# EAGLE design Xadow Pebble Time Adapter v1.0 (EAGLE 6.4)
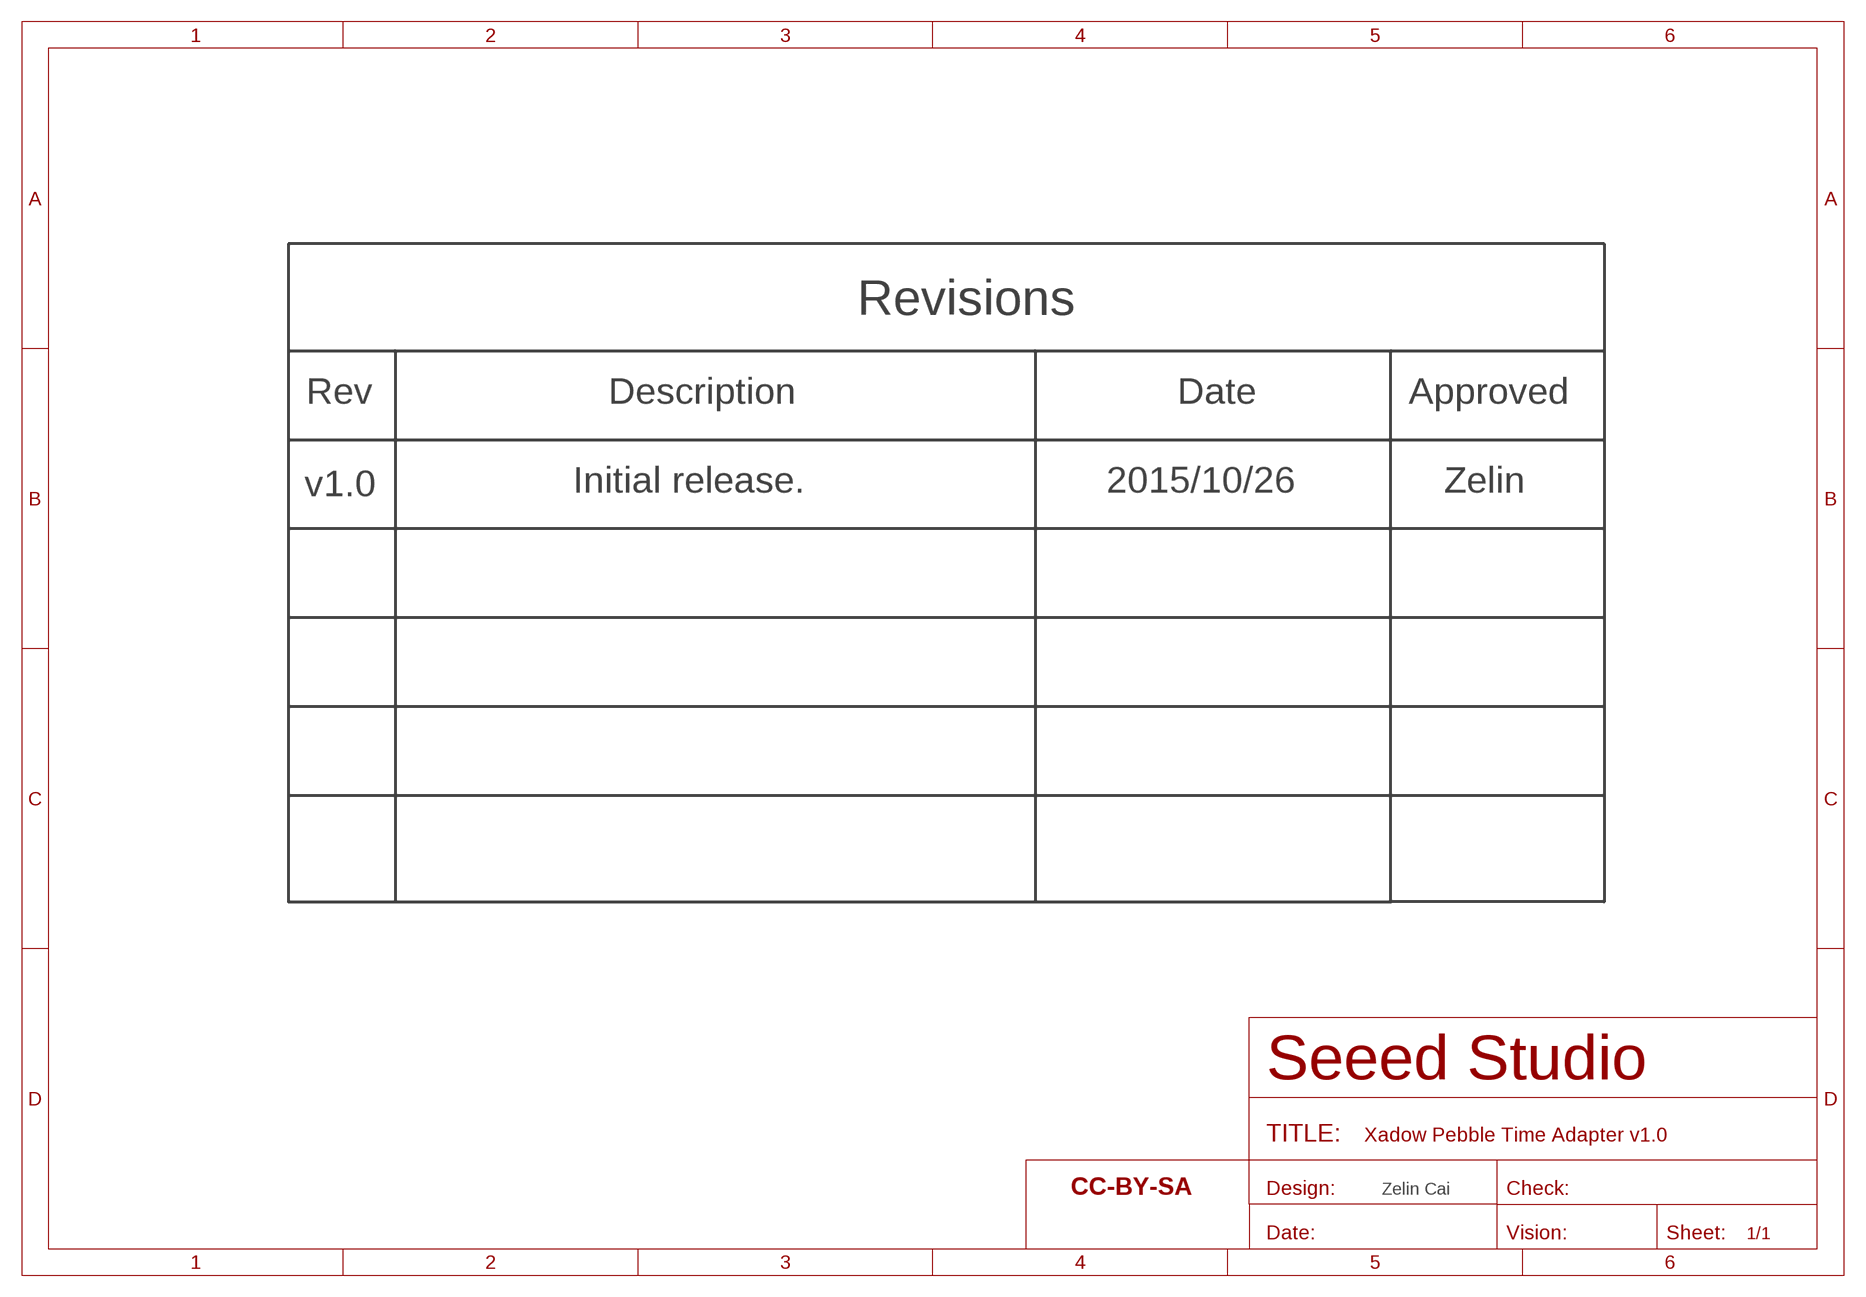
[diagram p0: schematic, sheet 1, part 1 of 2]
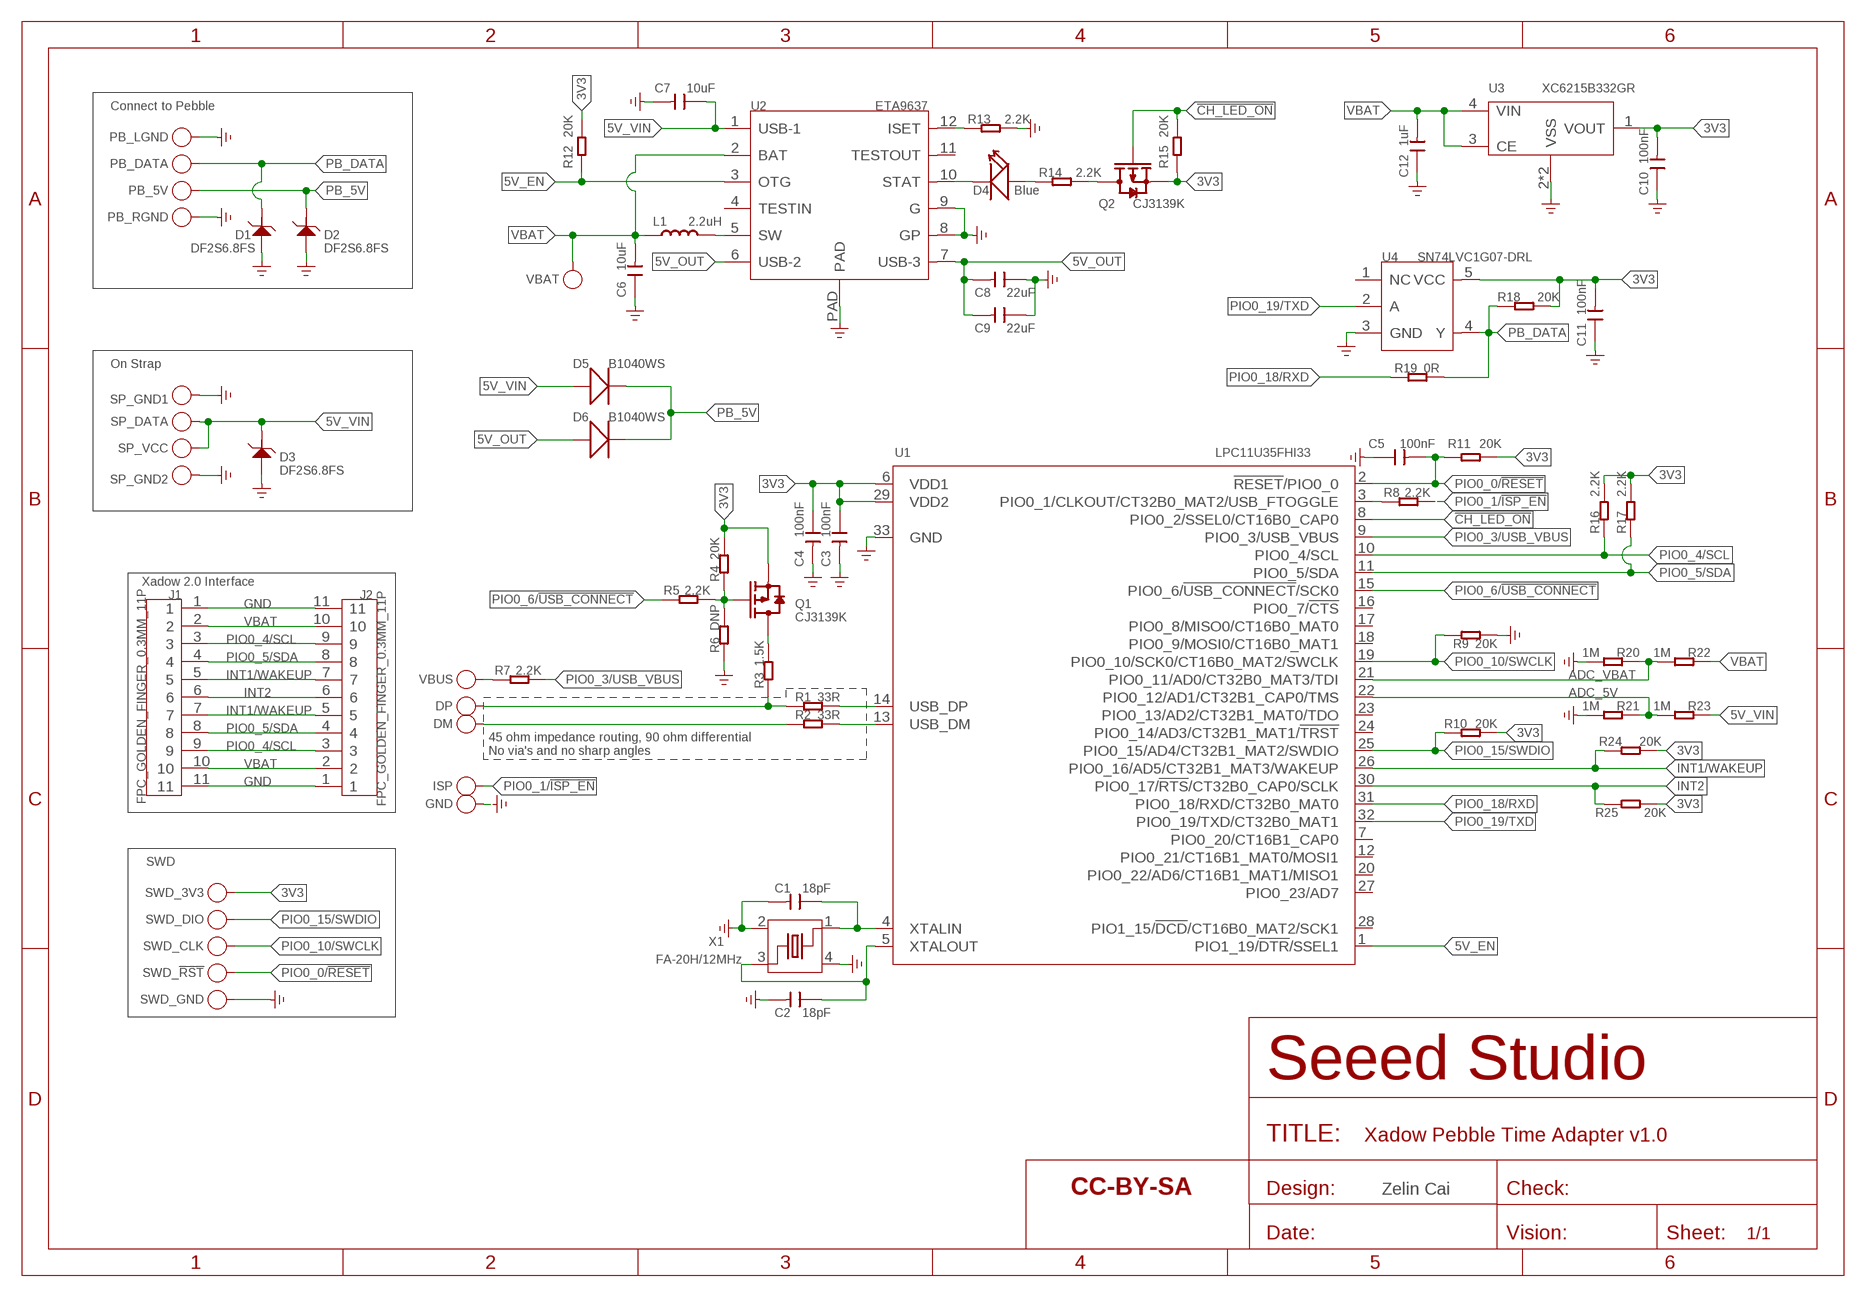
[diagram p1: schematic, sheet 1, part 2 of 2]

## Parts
C1  18pF  CAP-0201  [C0201]
C2  18pF  CAP-0201  [C0201]
C3  100nF  CAP-0201  [C0201]
C4  100nF  CAP-0201  [C0201]
C5  100nF  CAP-0201  [C0201]
C6  10uF  CAP-0805  [C0805]
C7  10uF  CAP-0805  [C0805]
C8  22uF  CAP-0805  [C0805]
C9  22uF  CAP-0805  [C0805]
C10  100nF  CAP-0201  [C0201]
C11  100nF  CAP-0201  [C0201]
C12  1uF  CAP-0402  [C0402]
D1  DF2S6.8FS  D-ESD-2P'DF2S6.8FS'  [SOD-923]
D2  DF2S6.8FS  D-ESD-2P'DF2S6.8FS'  [SOD-923]
D3  DF2S6.8FS  D-ESD-2P'DF2S6.8FS'  [SOD-923]
D4  Blue  LED'0402'  [LED-0402]
D5  B1040WS  DIODE'0805'  [SOD-323]
D6  B1040WS  DIODE'0805'  [SOD-323]
DM  DM  TEST-POINT'4545'  [TP-D45MIL]
DP  DP  TEST-POINT'4545'  [TP-D45MIL]
FR1  PAGE1  SEEEDSTUDIO-OPEN-SCH-FRAME  [SEEEDSTUDIO-PCB-FRAME]
FR2  PAGE2  SEEEDSTUDIO-OPEN-SCH-FRAME  [SEEEDSTUDIO-PCB-FRAME]
GND  GND  TEST-POINT'4545'  [TP-D45MIL]
ISP  ISP  TEST-POINT'4545'  [TP-D45MIL]
J1  FPC_GOLDEN_FINGER_0.3MM_11P  FPC-GOLDFINGER-11(FH35C-11S-0.3SHW(50))  [FPC_GOLDEN_FINGER_0.3MM_11P(FH35C-11S-0.3SHW(50))]
J2  FPC_GOLDEN_FINGER_0.3MM_11P  FPC-GOLDFINGER-11(FH35C-11S-0.3SHW(50))  [FPC_GOLDEN_FINGER_0.3MM_11P(FH35C-11S-0.3SHW(50))]
L1  2.2uH  INDUCTOR/FERRITE-BEAD'0806'  [L0806]
PB_5V  Pogo_M014  POGO-PIN-86  [TP-D86MIL$1]
PB_DATA  Pogo_M014  POGO-PIN-86  [TP-D86MIL$1]
PB_LGND  Pogo_M041  POGO-PIN-100  [TP-D100MIL]
PB_RGND  Pogo_M041  POGO-PIN-100  [TP-D100MIL]
Q1  CJ3139K  MOSFET-P-CJ3139K  [SOT-723]
Q2  CJ3139K  MOSFET-P-CJ3139K  [SOT-723]
R1  33R  RES-0201  [R0201]
R2  33R  RES-0201  [R0201]
R3  1.5K  RES-0201  [R0201]
R4  20K  RES-0201  [R0201]
R5  2.2K  RES-0201  [R0201]
R6  DNP  RES-0201  [R0201]
R7  2.2K  RES-0201  [R0201]
R8  2.2K  RES-0201  [R0201]
R9  20K  RES-0201  [R0201]
R10  20K  RES-0201  [R0201]
R11  20K  RES-0201  [R0201]
R12  20K  RES-0201  [R0201]
R13  2.2K  RES-0201  [R0201]
R14  2.2K  RES-0201  [R0201]
R15  20K  RES-0201  [R0201]
R16  2.2K  RES-0201  [R0201]
R17  2.2K  RES-0201  [R0201]
R18  20K  RES-0201  [R0201]
R19  0R  RES-0201  [R0201]
R20  1M  RES-0201  [R0201]
R21  1M  RES-0201  [R0201]
R22  1M  RES-0201  [R0201]
R23  1M  RES-0201  [R0201]
R24  20K  RES-0201  [R0201]
R25  20K  RES-0201  [R0201]
SP_DATA  5V_VIN  POGO-PIN-86  [TP-D86MIL$1]
SP_GND1  GND  POGO-PIN-1-2.0MM  [TP-D2.0MM]
SP_GND2  GND  POGO-PIN-1-2.0MM  [TP-D2.0MM]
SP_VCC  5V_VIN  POGO-PIN-86  [TP-D86MIL$1]
SWD_3V3  SWD_3V3  TEST-POINT'4545'  [TP-D45MIL]
SWD_!RST  SWD_!RST  TEST-POINT'4545'  [TP-D45MIL]
SWD_CLK  SWD_CLK  TEST-POINT'4545'  [TP-D45MIL]
SWD_DIO  SWD_DIO  TEST-POINT'4545'  [TP-D45MIL]
SWD_GND  SWD_GND  TEST-POINT'4545'  [TP-D45MIL]
U1  LPC11U35FHI33  MCU-LPC11U35FHI33/501  [QFN32G-0.5-5X5MM]
U2  ETA9637  PMIC-ETA9637  [QFN12-0.45-3X3MM]
U3  XC6215B332GR  PMIC-XC6215-3V3  [USP4-0.6-1.2X1.6MM]
U4  SN74LVC1G07-DRL  LOGIC-SN74LVC1G07-DRL  [5P-SDM-1.6X1.2X0.5MM]
VBAT  VBAT  TEST-POINT'4545'  [TP-D45MIL]
VBUS  VBUS  TEST-POINT'4545'  [TP-D45MIL]
X1  FA-20H/12MHz  CRYSTAL'NX2520SA'  [X4-SMD-2.5X2.0X0.8MM]

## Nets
3V3: C3.1 C4.1 C10.2 C11.2 Q1.3(S) Q2.3(S) R4.2 R10.2 R11.1 R12.2 R15.1 R16.1 R17.1 R18.2 R24.1 R25.2 SWD_3V3.T U1.6(VDD1) U1.29(VDD2) U3.1(VOUT) U4.5(VCC)
5V_EN: R12.1 U1.1(PIO1_19/!DTR!/SSEL1) U2.3(OTG)
5V_OUT: C8.2 C9.2 D6.+ U2.6(USB-2) U2.7(USB-3)
5V_VIN: C7.1 D3.1 D5.+ R23.1 SP_DATA.T SP_VCC.T U2.1(USB-1)
!CH_LED_ON: Q2.1(G) R15.2 U1.8(PIO0_2/SSEL0/CT16B0_CAP0)
ADC_5V: R21.1 R23.2 U1.22(PIO0_12/AD1/CT32B1_CAP0/TMS)
ADC_VBAT: R20.1 R22.2 U1.21(PIO0_11/AD0/CT32B0_MAT3/TDI)
GND: C1.2 C2.2 C3.2 C4.2 C5.1 C6.1 C7.2 C8.1 C9.1 C10.1 C11.1 C12.1 D1.2 D2.2 D3.2 GND.T J1.1 J1.11 J2.1 J2.11 PB_LGND.T PB_RGND.T R6.1 R9.2 R13.1 R20.2 R21.2 SP_GND1.T SP_GND2.T SWD_GND.T U1.33(GND) U2.8(GP) U2.9(G) U2.PAD U3.2(VSS) U3.PAD(VSS) U4.3(GND) X1.2 X1.4 ; supply symbol labelled GND_POWER
INT1/WAKEUP: J1.5 J1.7 J2.5 J2.7 R24.2 U1.26(PIO0_16/AD5/CT32B1_MAT3/WAKEUP)
INT2: J1.6 J2.6 R25.1 U1.30(PIO0_17/!RTS!/CT32B0_CAP0/SCLK)
N$1: C1.1 U1.4(XTALIN) X1.1
N$2: Q1.2(D) R3.2
N$3: C2.1 U1.5(XTALOUT) X1.3
N$4: R1.2 U1.14(USB_DP)
N$5: R2.2 U1.13(USB_DM)
N$6: DP.T R1.1 R3.1
N$7: Q1.1(G) R4.1 R5.1 R6.2
N$8: DM.T R2.1
N$9: R7.2 VBUS.T
N$10: R8.2 U1.3(PIO0_1/CLKOUT/CT32B0_MAT2/USB_FTOGGLE)
N$11: L1.2 U2.5(SW)
N$12: R13.2 U2.12(ISET)
N$13: D4.- U2.10(STAT)
N$14: D4.+ R14.2
N$15: Q2.2(D) R14.1
PB_5V: D2.1 D5.- D6.- PB_5V.T
PB_DATA: D1.1 PB_DATA.T R18.1 R19.1 U4.4(Y)
PIO0_0/!RESET: C5.2 R11.2 SWD_!RST.T U1.2(!RESET!/PIO0_0)
PIO0_1/!ISP_EN: ISP.T R8.1
PIO0_3/USB_VBUS: R7.1 U1.9(PIO0_3/USB_VBUS)
PIO0_4/SCL: J1.3 J1.9 J2.3 J2.9 R16.2 U1.10(PIO0_4/SCL)
PIO0_5/SDA: J1.4 J1.8 J2.4 J2.8 R17.2 U1.11(PIO0_5/SDA)
PIO0_6/!USB_CONNECT: R5.2 U1.15(PIO0_6/!USB_CONNECT!/SCK0)
PIO0_10/SWCLK: R9.1 SWD_CLK.T U1.19(PIO0_10/SCK0/CT16B0_MAT2/SWCLK)
PIO0_15/SWDIO: R10.1 SWD_DIO.T U1.25(PIO0_15/AD4/CT32B1_MAT2/SWDIO)
PIO0_18/RXD: R19.2 U1.31(PIO0_18/RXD/CT32B0_MAT0)
PIO0_19/TXD: U1.32(PIO0_19/TXD/CT32B0_MAT1) U4.2(A)
VBAT: C6.2 C12.2 J1.2 J1.10 J2.2 J2.10 L1.1 R22.1 U2.2(BAT) U3.3(CE) U3.4(VIN) VBAT.T
Unconnected: U1.7(PIO0_20/CT16B1_CAP0) U1.12(PIO0_21/CT16B1_MAT0/MOSI1) U1.16(PIO0_7/!CTS!) U1.17(PIO0_8/MISO0/CT16B0_MAT0) U1.18(PIO0_9/MOSI0/CT16B0_MAT1) U1.20(PIO0_22/AD6/CT16B1_MAT1/MISO1) U1.23(PIO0_13/AD2/CT32B1_MAT0/TDO) U1.24(PIO0_14/AD3/CT32B1_MAT1/!TRST!) U1.27(PIO0_23/AD7) U1.28(PIO1_15/!DCD!/CT16B0_MAT2/SCK1) U2.4(TESTIN) U2.11(TESTOUT) U4.1(NC)

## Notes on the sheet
- Connect to Pebble
- Revisions
- On Strap
- Rev | Description | Date | Approved
- v1.0 | Initial release. | 2015/10/26 | Zelin
- Xadow 2.0 Interface
- 45 ohm impedance routing, 90 ohm differential
  No via's and no sharp angles
- SWD
- Zelin Cai | Zelin Cai

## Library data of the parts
C1-C12 = Discrete-new:CAP: Ceramic Capacitors
D1-D3 = Discrete-new:D-ESD-2P: SOD-923:304060009;SOD-123:304060001
D4 = Discrete-new:LED
D5 D6 = Discrete-new:DIODE*
DM DP GND ISP SWD_3V3 SWD_!RST SWD_CLK SWD_DIO SWD_GND VBAT VBUS = Discrete-new:TEST-POINT; PARTNO: DNP
FR1 FR2 = moudle-new:SEEEDSTUDIO-OPEN-SCH-FRAME
J1 J2 = Connector:FPC-GOLDFINGER-11(FH35C-11S-0.3SHW(50))
L1 = Discrete-new:INDUCTOR/FERRITE-BEAD
PB_5V PB_DATA PB_LGND PB_RGND SP_DATA SP_VCC = Connector-new:POGO-PIN
Q1 Q2 = Discrete-new:MOSFET-P
R1-R25 = Discrete-new:RES
SP_GND1 SP_GND2 = Connector-new:POGO-PIN-1
U1 = IC-new:MCU-LPC11U35FHI33/501: 310010053
U2 = template:PMIC-ETA9637: 1.5A Linear Charger with 1A OTG
U3 = IC-new:PMIC-XC6215-3V3
U4 = template:LOGIC-SN74LVC1G07: SN74LVC1G07 Single Buffer/Driver With Open-Drain Output
X1 = Discrete-new:CRYSTAL

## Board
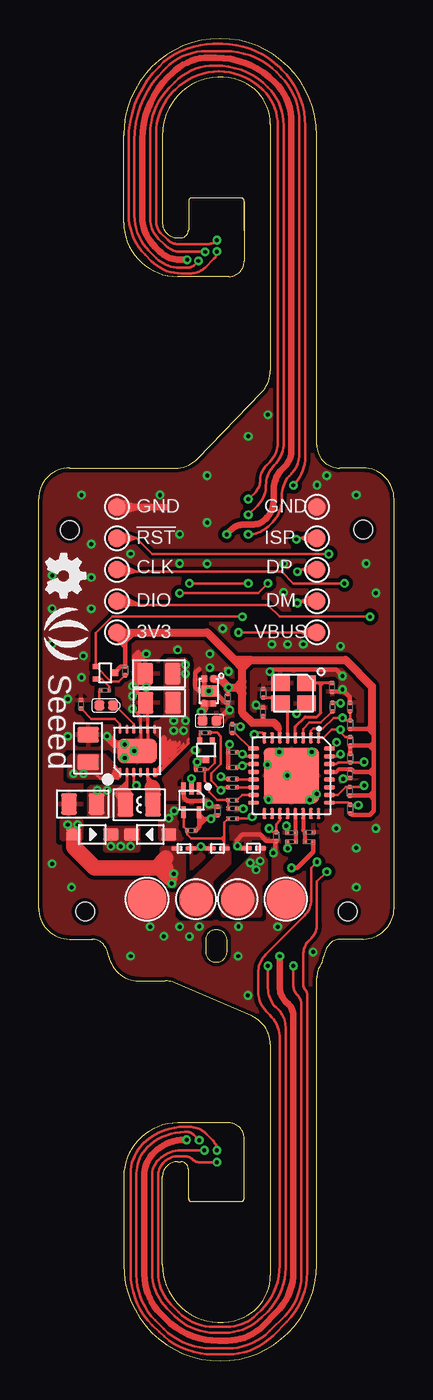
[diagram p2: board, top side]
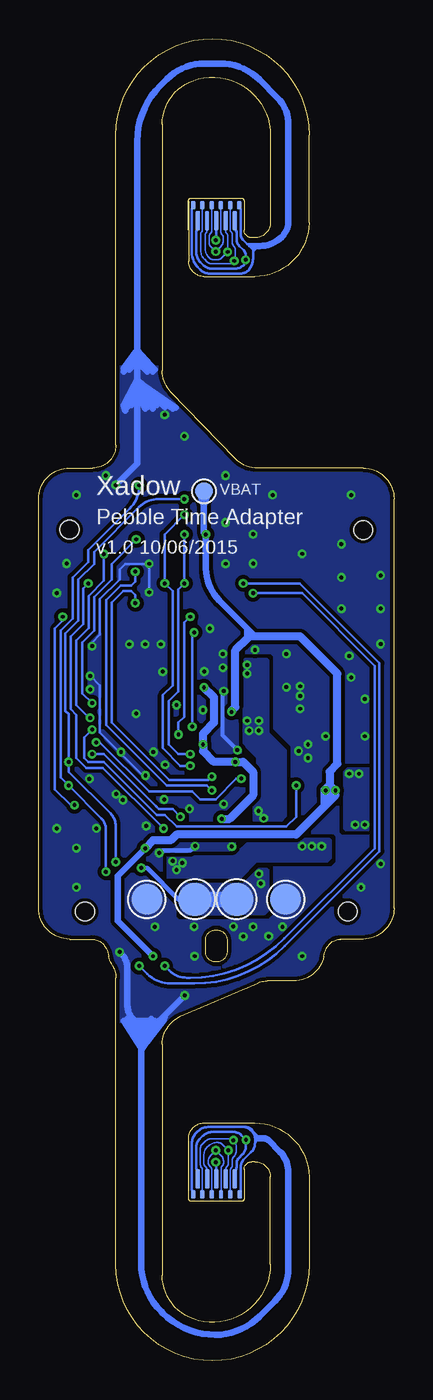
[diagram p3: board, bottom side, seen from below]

Size 23 x 85.6 mm. Coordinates in mm from the lower left corner, seen from the top.
Outline: 58 segments
Copper layers (1*16): Top 0.035mm / dielectric 1.5mm / Bottom 0.035mm
Design rules "SeeedStudio_2layer_DRU_no_angle_20140221 *": minimum track width 1mil, minimum drill 10mil, track to track 6mil, track to pad 6mil, pad to pad 6mil, via to via 6mil, smd to smd 0mil, copper to edge 10mil, drill to drill 10mil, minimum pad ring 10mil, minimum via ring 6mil, stop-mask expansion 2mil, vias tented up to drill 25mil, thermal gap 10mil
Holes 1.2 mm at 20,29.09 3,29.09 21,53.81 2,53.79
tRestrict: 1 lines

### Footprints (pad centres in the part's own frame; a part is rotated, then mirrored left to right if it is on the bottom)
C0201 = smd 0.279 x 0.318: 1 -0.279,0; 2 0.279,0
C0805 = smd 1.397 x 1.016: 1 0,0.889; 2 0,-0.889
C0402 = smd 0.635 x 0.635: 1 0,0.445; 2 0,-0.445
SOD-923 = smd 0.7 x 0.3: 1 -0.45,0; 2 0.45,0
LED-0402 = smd 0.635 x 0.635: + -0.445,0; - 0.445,0
SOD-323 = smd 1 x 0.8: + -1.2,0; - 1.2,0
TP-D45MIL = smd 1.143 x 1.143: T 0,0
FPC_GOLDEN_FINGER_0.3MM_11P(FH35C-11S-0.3SHW(50)) = smd 0.28 x 0.55: 1 -1.5,0; 3 -0.9,0; 5 -0.3,0; 7 0.3,0; 9 0.9,0; 11 1.5,0 | smd 0.28 x 1.25: 2 -1.2,-1; 4 -0.6,-1; 6 0,-1; 8 0.6,-1; 10 1.2,-1
L0806 = smd 1.016 x 1.524: 1 -0.889,0; 2 0.889,0
TP-D86MIL$1 = smd 2.184 x 2.184: T 0,0
TP-D100MIL = smd 2.54 x 2.54: T 0,0
SOT-723 = smd 0.32 x 0.4: 1 -0.4,-0.6; 2 0.4,-0.6 | smd 0.42 x 0.5: 3 0,0.6
R0201 = smd 0.279 x 0.318: 1 -0.279,0; 2 0.279,0
TP-D2.0MM = smd 2 x 2: T 0,0
QFN32G-0.5-5X5MM = smd 0.7 x 0.25: 1 -2.45,1.75; 2 -2.45,1.25; 3 -2.45,0.75; 4 -2.45,0.25; 5 -2.45,-0.25; 6 -2.45,-0.75; 7 -2.45,-1.25; 8 -2.45,-1.75; 17 2.45,-1.75; 18 2.45,-1.25; 19 2.45,-0.75; 20 2.45,-0.25; 21 2.45,0.25; 22 2.45,0.75; 23 2.45,1.25; 24 2.45,1.75 | smd 0.25 x 0.7: 9 -1.75,-2.45; 10 -1.25,-2.45; 11 -0.75,-2.45; 12 -0.25,-2.45; 13 0.25,-2.45; 14 0.75,-2.45; 15 1.25,-2.45; 16 1.75,-2.45; 25 1.75,2.45; 26 1.25,2.45; 27 0.75,2.45; 28 0.25,2.45; 29 -0.25,2.45; 30 -0.75,2.45; 31 -1.25,2.45; 32 -1.75,2.45 | smd 3.6 x 3.6: 33 0,0
QFN12-0.45-3X3MM = smd 0.2 x 0.6: 1 -1.125,-1.4; 2 -0.675,-1.4; 3 -0.225,-1.4; 4 0.225,-1.4; 5 0.675,-1.4; 6 1.125,-1.4; 7 1.125,1.4; 8 0.675,1.4; 9 0.225,1.4; 10 -0.225,1.4; 11 -0.675,1.4; 12 -1.125,1.4 | smd 2.55 x 1.6: PAD 0,0
USP4-0.6-1.2X1.6MM = smd 0.36 x 0.4: 1 -0.3,-0.8; 2 0.3,-0.8; 3 0.3,0.8; 4 -0.3,0.8 | smd 1 x 0.7: PAD 0,0
5P-SDM-1.6X1.2X0.5MM = smd 0.3 x 0.75: 1 -0.5,-0.775; 2 0,-0.775; 3 0.5,-0.775; 4 0.5,0.775; 5 -0.5,0.775
X4-SMD-2.5X2.0X0.8MM = smd 1.2 x 1: 1 -0.85,-0.65; 2 0.85,-0.65; 3 0.85,0.65; 4 -0.85,0.65

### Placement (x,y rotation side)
C1  18.99,43.6 270 top
C2  14.53,43.22 90 top
C3  20.15,38.01 270 top
C4  14.52,42.01 90 top
C5  20.15,42.33 270 top
C6  2.85,36.04 90 top
C7  3.21,39.65 180 top
C8  7.8,42.61 90 top
C9  7.79,44.49 90 top
C10  12.24,42.9 90 top
C11  11.59,35.6 270 top
C12  11.05,41.44 270 top
D1  11.58,33.18 180 top
D2  13.9,33.18 180 top
D3  9.41,33.17 0 top
D4  4.37,42.43 0 top
D5  3.47,34.07 0 top
D6  7.22,34.07 180 top
DM  18.01,49.19 0 top
DP  18.01,51.22 0 top
FR1  not placed on the board
FR2  not placed on the board
GND  18.01,55.28 0 top
ISP  18.01,53.25 0 top
J1  11.5,74.81 0 bottom
J2  11.5,10.79 180 bottom
L1  6.51,36 0 top
PB_5V  12.88,29.88 0 top
PB_DATA  10.19,29.88 0 top
PB_LGND  7.02,29.88 0 top
PB_RGND  15.99,29.88 0 top
Q1  10.84,39.55 180 top
Q2  4.31,44.54 270 top
R1  12.55,37.14 0 top
R2  12.55,37.67 0 top
R3  10.77,40.67 180 top
R4  10.46,38.29 180 top
R5  12.55,36.3 0 top
R6  12.55,35.76 180 top
R7  12.53,40.93 90 top
R8  19.02,42.33 270 top
R9  15.37,33.95 270 top
R10  20.16,35.73 270 top
R11  20.16,41.19 90 top
R12  20.17,40.11 270 top
R13  2.74,42.51 270 top
R14  4.28,43.41 180 top
R15  5.61,44.67 270 top
R16  12.55,39.41 0 top
R17  12.55,38.42 0 top
R18  9.89,34.34 0 top
R19  12.55,35.1 0 top
R20  16.36,34.2 180 top
R21  17.51,34.23 0 top
R22  16.36,33.62 0 top
R23  17.51,33.62 180 top
R24  20.13,36.87 90 top
R25  20.17,39.03 90 top
SP_DATA  10.19,29.88 0 bottom
SP_GND1  7.02,29.88 0 bottom
SP_GND2  15.99,29.88 0 bottom
SP_VCC  12.88,29.88 0 bottom
SWD_3V3  5.06,47.16 180 top
SWD_!RST  5.06,53.25 180 top
SWD_CLK  5.06,51.22 180 top
SWD_DIO  5.06,49.19 180 top
SWD_GND  5.06,55.28 180 top
U1  16.36,37.88 270 top
U2  6.38,39.48 0 top
U3  11.02,43.36 180 top
U4  9.89,36.28 180 top
U$32  [SEEED-SILK-160*153MIL]  1.88,47.03 270 top
U$33  [OSHW_FILLX100_NOTEXT]  0.49,52.24 270 top
VBAT  12.3,56.3 90 bottom
VBUS  18.01,47.16 0 top
X1  16.49,43.22 180 top

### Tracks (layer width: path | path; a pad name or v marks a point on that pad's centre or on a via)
3V3  (via drill 0.25 pad 0.51)
  Top 0.152: 21.57,41.06 21.51,41.12
  Top 0.254: U1.6 15.61,40.92 15.47,41.06 | 14.46,41.31 14.52,41.38 C4.1 14.52,41.63 | 14.52,41.63 14.33,41.44 | 14.52,41.63 14.71,41.44 | U1.29 19.28,38.13 19.44,38.29 C3.1
  Top 0.305: C10.2 12.24,43.54 v12.3,43.6 | U4.5 10.39,35.1 | R4.2 10.18,38.68 v10.27,38.77 10.44,38.95 Q1.3 | R10.2 20.2,35.45 20.3,35.34 21.44,35.34 21.7,35.6 21.7,36.36 | 21.7,36.36 21.7,36.61 | 21.7,36.61 21.7,36.87 | 21.7,36.87 21.7,37.88 | 21.7,37.88 21.7,38.14 | 21.7,38.14 21.7,38.39 | 21.7,38.39 21.7,39.54 | 21.7,39.54 21.7,39.79 | R11.1 21.33,40.91 | 21.34,40.91 21.67,40.91 21.7,40.93 | 21.4,39.83 R12.2 R25.2 | 21.48,39.83 21.66,39.83 21.7,39.79 | C3.1 20.27,38.29 20.43,38.14 21.44,38.14 | 21.44,38.14 21.7,38.14 | R17.1 R16.1 12.27,39.83 v12.36,39.92 | R24.1 21.42,36.59 | 21.47,36.59 21.67,36.59 21.7,36.61 | 21.7,39.79 21.7,40.04 | 21.7,40.04 21.7,40.55 | 21.7,40.55 21.7,40.93 | 21.7,40.93 21.7,41.19 | 21.33,40.91 21.33,40.94 21.51,41.12 21.57,41.19 | 21.33,40.91 21.34,40.91 | 21.34,40.91 21.7,40.55 | 21.4,39.83 21.48,39.83 | 21.48,39.83 21.7,40.04 | 21.4,39.83 21.7,39.54 | 21.44,38.14 21.7,38.39 | 21.44,38.14 21.7,37.88 | 21.42,36.59 21.7,36.87 | 21.42,36.59 21.47,36.59 | 21.47,36.59 21.7,36.36 | C11.2 11.38,35.32 v11.16,35.09 10.77,35.09 | 10.55,34.86 10.55,34.94 10.39,35.09 | 10.65,35.09 10.39,35.09 | 10.39,35.09 10.39,35.1 | 10.77,35.09 10.65,35.09 | 10.65,35.09 10.39,35.34 | 10.77,35.09 10.55,34.86 | 10.39,35.1 10.39,34.56 R18.2 | 10.55,34.86 10.39,34.71 | 5.61,46.23 R15.1 5.32,44.95 Q2.3 | 5.61,46.23 5.61,46.52 | 5.61,46.56 5.61,47.12 5.57,47.16 | 5.61,46.52 5.56,46.52 5.19,46.9 | 5.61,46.52 5.61,46.56 | 5.61,46.56 6.08,47.03 5.19,47.54 | 5.61,46.23 4.93,46.9
  Top 0.508: 12.22,43.52 v12.3,43.6 | v12.3,43.6 12.81,43.6 | 12.81,43.6 13.19,43.6 | 15.47,41.06 15.22,41.31 14.46,41.31 13.82,41.31 13.19,41.95 13.19,43.22 | U3.1 11.74,44.16 v12.3,43.6 | 13.19,43.22 13.19,43.6 | 13.19,43.6 13.19,43.98 | 12.81,43.6 13.19,43.98 | 12.81,43.6 13.19,43.22 | 13.7,45.38 19.86,45.38 21.57,43.67 21.57,41.06 | 13.7,45.38 13.19,45.38 | 13.19,45.38 12.68,45.38 | 13.19,43.98 13.19,44.87 | 13.19,44.87 13.19,45.38 | 13.19,44.87 12.68,45.38 | 13.19,44.87 13.7,45.38 | 12.68,45.38 10.9,47.16 5.57,47.16 SWD_3V3.T
  Bottom 0.508: v12.3,43.6 11.66,42.96 11.66,41.31 12.36,40.61 v12.36,39.92 12.36,39.47 11.66,38.77 v10.27,38.77 9.76,38.77 9.12,38.14 9.12,36.61 10.65,35.09 v11.16,35.09
5V_EN  (via drill 0.25 pad 0.51)
  Top 0.152: U2.3 6.16,37.42 v6.33,37.25 | U1.1 18.43,40.33 18.97,40.87 v19.54,40.87 19.54,40.68 19.83,40.39 R12.1
  Bottom 0.152: v19.54,40.87 20.05,40.36 20.05,39.03 19.79,38.77 18.78,38.77 15.35,35.34 14.84,35.34 14.08,34.58 6.96,34.58 6.33,35.22 v6.33,37.25
5V_OUT  (via drill 0.25 pad 0.51)
  Top 0.203: 8.23,38.9 8.11,38.77 7.51,38.17 U2.6 7.67,38.08 | 8.23,38.9 8.49,39.15 8.49,40.17 | 7.67,38.08 8.49,38.9 | 7.67,38.08 7.6,38.01 7.54,38.01 | 8.49,38.9 8.49,38.77 | 8.49,38.77 7.6,37.88 7.54,37.88 | 8.49,38.9 8.62,39.03 | 8.62,39.03 8.74,39.15 | 8.74,39.15 8.74,40.04 | 8.49,38.77 8.87,39.15 | 8.87,39.15 8.87,39.41 | 8.87,39.66 8.87,39.79 | 8.87,39.79 8.87,40.04 | 8.62,39.03 8.62,39.66 | 8.62,39.66 8.62,40.04 | 8.62,39.66 8.36,39.92 | 8.87,39.79 9.12,40.04 | 8.23,38.9 8.36,38.9 8.36,40.04 | 8.74,39.15 8.87,39.15 | 8.87,39.15 9.7,39.98 9.7,40.23 | 8.87,39.41 9.38,39.92 | 8.87,39.41 8.87,39.66 | 8.87,39.66 9.12,39.92
  Top 0.406: 8.11,38.77 8.11,40.3
  other vias: 9.5,45.06 9.5,44.49 8.43,35.13 8.77,35.6 9.5,41.44 8.74,41.44 8.74,40.81 9.38,40.81
  pour Top (isolate 0.254, no thermals): 8.11,33.69 9.25,33.69 9.38,33.82 9.38,35.85 9.25,35.98 7.85,35.98 7.73,35.85 7.73,33.82 7.85,33.69
  pour Top (isolate 0.254, no thermals): 7.41,40.74 7.41,40.55 8.11,39.85 9.44,39.85 9.76,40.17 9.76,45.25 9.5,45.5 8.36,45.5 8.11,45.25 8.11,41.82 7.73,41.44 7.54,41.44 7.41,41.31
  pour Bottom (isolate 0.254, no thermals): 6.96,39.54 6.96,35.24 7.37,34.84 9,34.84 9.12,34.96 9.12,36.11 8.87,36.36 8.87,39.03 9.76,39.92 9.76,45.38 9.63,45.5 8.23,45.5 8.11,45.38 8.11,40.68
5V_VIN  (via drill 0.25 pad 0.51)
  Top 0.203: U2.1 5.26,37.83 5.12,37.69 3.98,37.69 3.79,37.88 | U2.1 5.26,37.95 5.06,37.76 4.81,37.76 | U2.1 5.06,37.88 4.81,37.88 | U2.1 4.88,38.08 | 4.88,38.08 4.81,38.01 | 4.88,38.08 4.93,38.14 5.19,38.14 4.93,38.39 | 4.88,38.08 4.88,38.21 4.93,38.27 5.19,38.27 4.93,38.52
  Top 0.305: R23.1 17.78,32.96 16.74,31.92 v16.36,31.92
  Top 1.016: 7.6,31.92 3.64,31.92 2.27,33.28 D5.+ | 7.6,31.92 8.23,31.92 | 7.6,31.92 8.23,32.55 | 6.84,31.92 7.85,31.92 8.49,31.28
  Bottom 0.305: SP_VCC.T 13.95,29.88 15.98,31.92 v16.36,31.92
  Bottom 1.016: SP_VCC.T SP_DATA.T 10.19,30.02
  other vias: 8.62,30.9 8.74,31.53 2.9,38.01 2.27,38.01 2.52,34.71 1.88,34.71
  pour Top (isolate 0.254, no thermals): 4.81,37.63 2.06,37.63 1.88,37.81 1.88,39.1 2.06,39.28 4.3,39.28 4.93,38.65 4.93,37.76
  pour Bottom (isolate 0.254, no thermals): 9.89,30.9 13.57,30.9 13.82,30.65 13.82,28.99 13.7,28.87 9.89,28.87 9.76,28.99 9.76,30.77
  pour Bottom (isolate 0.254, no thermals): 11.28,28.87 9.76,30.9 11.28,30.9 11.41,30.77 11.41,28.99
  pour Bottom (isolate 0.254, no thermals): 9.76,30.9 8.87,31.79 8.74,31.92 8.23,31.92 8.11,31.79 8.11,29.12 8.36,28.87 11.03,28.87 11.16,28.99 11.16,30.77 11.03,30.9
  pour Top (isolate 0.254, no thermals): 7.98,30.65 8.87,30.65 9.5,31.28 9.5,33.19 9.38,33.31 7.98,33.31 7.85,33.19 7.85,30.77
  pour Top (isolate 0.254, no thermals): 1.88,33.69 2.77,33.69 2.9,33.82 2.9,34.96 2.77,35.09 1.5,35.09 1.38,34.96 1.38,33.82 1.5,33.69
  pour Bottom (isolate 0.254, no thermals): 2.39,34.33 1.63,34.33 1.5,34.46 1.5,38.27 1.63,38.39 3.03,38.39 3.28,38.14 3.28,34.46 3.15,34.33
!CH_LED_ON  (via drill 0.25 pad 0.51)
  Top 0.152: U1.8 14.61,40.52 14.46,40.68 14.08,40.68 v13.95,40.55 | 3.73,45.07 3.73,45.05 3.72,45.04 Q2.1 | v13.19,48.17 4.75,48.17 3.71,47.13 Q2.1 | R15.2 5.59,44.39 5.19,43.98 4.68,43.98 Q2.1
  Bottom 0.152: v13.95,40.55 13.95,41.31 13.57,41.69 13.57,47.79 v13.19,48.17
ADC_5V
  Top 0.254: U1.22 17.11,34.34 R21.1 R23.2
ADC_VBAT
  Top 0.254: U1.21 16.61,34.23 R20.1 R22.2
GND  (via drill 0.25 pad 0.51)
  Top 0.203: v6.18,39.48 6.61,39.91 U2.9 6.61,41.69 v6.08,42.22 | U2.PAD 6.53,39.48 7.06,40.01 U2.8 7.06,42.47 C8.1
  Top 0.305: R6.1 13.21,35.76 v13.24,35.74 | C11.1 11.19,35.88 v11.03,36.04 10.84,36.23 9.63,36.23 9.39,36.48 U4.3 | C12.1 11.54,41.44 12.17,42.08 12.3,42.08 v12.36,42.14 12.24,42.27 C10.1 12.08,42.62 11.35,43.36 U3.PAD | 10.72,44.19 U3.2 10.72,43.66 U3.PAD | C5.1 20.15,42.99 v19.66,43.47 19.51,43.32 C1.2 | X1.2 15.64,43.94 v14.97,44.62 15.09,44.74 19.26,44.74 v19.66,44.34 | X1.4 17.34,42.54 v16.69,41.9 | R20.2 16.08,34.58 v16.03,34.63 | C3.2 19.77,37.73 v19.72,37.68 | C4.2 14.24,42.29 v14.08,42.46 | 12.12,44.79 v12.29,44.63 | U3.PAD 10.38,43.36 10.14,43.6 10.14,44.55 10.39,44.81 | v15.19,32.88 15.32,33.01 15.32,33.67 R9.2 14.74,33.67 14.33,34.07 13.19,34.07 12.81,33.69 12.81,33.39 v12.87,33.32 13.01,33.18 D2.2 | D3.2 10.38,33.17 v10.5,33.3 10.62,33.18 D1.2 | v6.08,43.68 6.08,43.73 6.2,43.85 6.2,45.01 | 6.2,45.01 6.35,45.15 | 6.35,45.15 v6.96,45.77 | 6.35,45.15 6.35,43.31 v6.08,43.04 | 6.2,45.01 6.2,45.63 6.46,45.89 | 6.35,45.15 6.35,45.52 6.58,45.76
  Top 0.406: 8.23,55.28 6.33,55.28 | 6.33,55.28 6.2,55.28 | 6.2,55.28 SWD_GND.T | v16.08,37.9 16.78,37.9 v17.99,36.69 | 5.55,39.9 v5.57,39.92 | 6.2,55.28 5.06,55.66 | 6.33,55.28 5.19,54.9 | v16.08,37.9 16.35,37.9 U1.33 | v16.08,37.9 16.08,37.55 v14.88,36.34
  Top 0.508: v5.57,39.92 4.95,39.92 v4.42,40.44
  Bottom 0.152: v16.08,37.9 16.25,37.9 19.03,40.68 19.03,43.73 19.66,44.36 | v19.54,46.27 19.54,46.52 19.03,47.03 19.03,49.31 17.76,50.58 17.76,51.22 17.38,51.6 v15.85,51.6 v15.85,49.76 | J1.1 13,74.64 13.09,74.56 13.09,71.73 arc-45 12.7,70.8 12.54,70.63 arc-45 11.96,70.4 9.89,70.4 arc-45 9.45,70.58 arc-45 9.12,71.36 9.12,71.79 | J1.11 10,74.65 9.91,74.56 9.91,72.88 arc-45 9.79,72.59 9.5,72.3 | 9.5,72.3 9.38,72.17 | 9.38,72.17 9.12,71.92 | 9.12,71.79 9.12,71.92 | 9.12,71.92 9,72.05 | 9.38,72.17 9.12,72.17 | 9.5,72.3 9.12,72.3 | 9.12,71.79 8.87,72.05 | J2.1 10,10.93 9.91,11.01 9.91,12.62 arc45 9.75,13 9.26,13.49 arc-45 9,14.12 9,14.14 | 9.84,15.15 11.93,15.15 arc-45 12.78,14.8 arc-45 13.09,14.05 13.09,11.14 arc-45 13,10.92 J2.11 | 9.84,15.15 arc45 9.27,14.92 9.15,14.8 | 9.15,14.8 arc45 9,14.42 | 9,14.42 9,14.14 | 9,14.42 8.77,14.42 | 9.15,14.8 8.74,14.39 8.74,14.52 9.16,14.93 arc-45 9.68,15.15 9.84,15.15 | 9,14.14 8.87,14.26
  Bottom 0.254: v10.14,39.54 11.09,40.49 11.09,43.28 U3.PAD
  Bottom 0.305: v12.87,33.32 12.92,33.32 13.19,33.06 15.02,33.06 v15.2,32.88
  Bottom 0.406: 8.77,14.42 8.49,14.42 arc45 8.11,14.26 7.39,13.55 arc45 6.84,12.21 6.84,5.99 arc45 7.72,3.85 8.69,2.89 arc45 11.58,1.69 arc45 14.97,3.1 15.08,3.2 arc45 16.36,6.3 16.36,20.1 | 16.36,20.1 16.36,20.23 | 16.36,20.23 16.36,20.61 | 16.36,20.61 16.36,20.84 | 16.36,20.84 v13.54,23.66 | 16.36,20.84 16.36,21.25 | 16.36,21.25 16.36,21.5 | 16.36,21.5 16.36,21.63 16.93,22.2 arc45 17.25,22.97 17.25,25.38 arc-45 17.66,26.37 v17.76,26.47 | 16.36,21.25 16.87,21.76 | 16.87,21.76 17.25,22.14 | 16.36,21.25 16.24,21.25 15.47,22.01 16.87,22.01 | 16.36,21.5 15.73,22.14 | 16.87,21.76 15.47,21.76 15.35,21.88 | v18.01,56.69 18,56.69 16.62,58.08 16.62,62.9 | 16.62,65.44 16.62,78.96 arc45 15.13,82.55 14.71,82.97 arc45 12.26,83.99 11.26,83.99 arc45 8.7,82.93 7.55,81.78 arc45 6.84,80.05 6.84,73.8 arc45 7.27,72.76 arc45 8.69,72.17 9.12,72.17 | 16.62,65.44 16.62,65.06 | 16.62,64.68 16.62,63.54 | 16.62,63.54 16.62,63.28 | 16.62,63.28 16.62,62.9 | 16.62,63.28 16.49,63.16 | 16.49,63.16 16.36,63.03 | 16.36,63.03 16.24,62.9 | 16.24,62.9 15.98,62.65 | 16.62,63.54 16.24,63.16 | 16.24,63.16 14.84,61.76 | 16.49,63.16 14.33,61.63 | 16.24,63.16 14.14,61.7 | 16.24,62.9 15.35,61.89 | 16.36,63.03 15.88,62.15 | 15.88,62.15 15.6,61.63 | 16.62,62.9 16.11,61.63 | 15.88,62.15 15.98,61.76 | 16.62,63.54 16.82,63.17 | 16.82,63.17 17.51,61.89 17.38,61.51 | 16.82,63.17 16.95,62.23 | 16.95,62.23 17,61.89 | 16.95,62.23 17.25,61.76 | 16.36,20.23 17.51,22.01 | 16.36,20.61 17,21.76 | 16.36,20.1 16.2,20.38 | 16.2,20.38 15.22,22.01 | 16.2,20.38 16,20.65 | 16,20.65 14.84,22.26 | 16,20.65 14.9,22.07 | 16.62,65.06 15.6,64.05 | 16.62,64.68 15.98,64.05 | 16.62,64.94 16.62,64.68 | 16.62,64.68 17.12,64.17
  Bottom 0.406: 16.62,65.06 16.62,64.94 | 16.62,64.94 17.51,64.05 | 16.62,65.44 17.51,64.24 | 16.62,65.44 15.47,64.17
  other vias: 5.57,39.03 7.22,28.11 15.47,28.11 11.02,43.36 15.09,46.39 19.26,34.48 10.9,54.27 10.9,51.6 2.14,30.66 0.87,46.41 0.87,48.69 0.87,50.85 7.85,56.06 20.55,56.06 20.55,30.66 20.55,33.2 2.77,56.06 10.39,28.12 12.93,28.12 21.19,51.61 21.82,49.71 12.91,26.2 14.81,38.6 15.58,39.42 17.54,36.31 17.67,39.42 8.11,27.48 9.76,27.47 9.12,28.11 0.87,32.18 21.82,34.47 10.9,57.32 13.57,59.86 14.84,61.25 18.65,57.32 5.95,26.2 6.96,43.61 1.88,40.44 1.88,42.85 2.77,44.25 9.12,51.61 2.9,45.64 3.41,50.72 3.41,48.69 3.41,52.88 5.95,52.25 9.12,53.52 11.08,44.88 11.08,45.77 9,46.03 16.11,46.39 17.12,46.39 11.92,47.41
  pour Bottom (isolate 0.254, rank 6): -0.02,64.3 23.09,64.3 23.09,22.01 -0.02,22.01
  pour Top (isolate 0.254, rank 6): -0.02,62.9 23.09,62.9 23.09,22.01 -0.02,22.01
INT1/WAKEUP  (via drill 0.25 pad 0.51)
  Top 0.152: U1.26 19.35,36.63 19.86,37.15 R24.2 20.96,37.15 v21.06,37.25 | v11.54,71.82 arc-45 11.34,71.34 10.78,70.78 arc-45 9.84,70.4 9.25,70.4 arc-45 7.3,71.2 6.91,71.6 arc-45 5.82,74.22 5.82,79.04 arc-45 7.79,83.8 arc-45 11.31,85.26 11.88,85.26 arc-45 15.63,83.7 15.75,83.59 arc-45 17.25,79.95 17.25,58.52 arc-45 v16.49,56.68 | v11.54,13.63 arc45 11.27,14.28 10.85,14.7 arc45 9.75,15.15 9.42,15.15 arc45 6.75,14.05 arc45 5.95,12.12 5.95,5.7 arc45 7.35,2.32 7.8,1.87 arc45 11.31,0.42 12.22,0.42 arc45 15.17,1.64 16.05,2.52 arc45 17.38,5.73 17.38,23.71 arc45 17.24,24.06 arc-45 17.12,24.33 17.12,26.29 arc-45 17.51,27.22 17.65,27.36 arc45 18.01,28.24 18.01,31.03 v18.65,31.66
  Bottom 0.102: J1.5 11.8,73.15 arc45 11.87,72.98 arc-45 11.97,72.75 11.97,72.38 arc-45 11.88,72.16 v11.54,71.82 11.2,72.16 arc-45 11.05,72.5 11.05,72.74 arc-45 11.12,72.9 arc45 11.2,73.1 J1.7 | J2.5 11.2,12.42 arc45 11.11,12.63 11.1,12.64 arc-45 11.03,12.82 11.03,12.9 arc-45 11.18,13.27 v11.54,13.63 11.88,13.29 arc-45 12.02,12.94 12.02,12.81 arc-45 11.95,12.65 11.88,12.57 arc45 11.8,12.37 J2.7
  Bottom 0.152: v18.65,31.66 18.65,34.44 arc-45 18.93,35.12 v21.06,37.25 21.57,37.76 21.57,47.28 20.81,48.04 20.81,50.71 19.79,51.73 19.79,52.49 17.12,55.16 arc-45 v16.49,56.68
INT2  (via drill 0.25 pad 0.51)
  Top 0.152: U1.30 19.27,38.63 19.39,38.75 R25.1 21.04,38.75 v21.06,38.77 | v11.54,72.56 11.5,72.52 arc-45 10.98,72.3 8.99,72.3 arc-45 8.35,72.57 7.9,73.02 arc-45 7.6,73.74 7.6,79.47 arc-45 8.73,82.19 8.84,82.31 arc-45 11.67,83.48 arc-45 14.48,82.31 14.54,82.26 arc-45 15.47,79.99 15.47,59.44 arc-45 14.96,58.2 14.75,57.99 arc45 14.33,56.97 arc-45 14.04,56.26 v13.57,55.79 | v11.54,12.87 10.37,12.87 arc-45 9.98,13.03 arc45 9.45,13.25 9.03,13.25 arc45 8.11,12.86 arc45 7.73,11.95 7.73,5.7 arc45 8.59,3.62 9.06,3.15 arc45 11.35,2.2 12.16,2.2 arc45 14.13,3.01 14.4,3.29 arc45 15.6,6.18 15.6,20.86 arc45 14.97,22.39 14.73,22.63 arc-45 14.2,23.89 14.2,25.13 arc-45 14.69,26.3 17.22,28.83 arc45 17.63,29.84 17.63,31.92 v18.01,32.3
  Bottom 0.152: v18.01,32.3 18.01,34.62 arc-45 18.35,35.42 21.06,38.14 v21.06,38.77 21.06,41.87 21.26,42.08 21.26,47.08 20.43,47.92 20.43,50.58 19.41,51.6 19.41,52.36 16.51,55.27 arc45 15.24,55.79 v13.57,55.79 | J1.6 11.5,72.59 v11.54,72.56 | J2.6 11.5,12.77 arc-45 v11.54,12.87
N$1
  Top 0.203: U1.4 16.61,41.06 17.25,41.69 18.01,41.69 18.27,41.95 18.27,43.73 | 18.27,43.73 18.27,43.88 | C1.1 18.27,43.88 | 18.27,43.88 17.35,43.88 X1.1 | 18.27,43.73 18.14,43.85 | 18.27,43.73 18.39,43.85
N$2
  Top 0.152: Q1.2 10.44,40.61 R3.2
N$3
  Top 0.203: U1.5 16.11,42.1 X1.3 15.27,42.94 C2.1
N$4
  Top 0.152: U1.14 R1.2
N$5
  Top 0.152: U1.13 12.87,37.63 R2.2
N$6  (via drill 0.25 pad 0.51)
  Top 0.152: R1.1 11.99,37.14 v11.79,36.93 11.16,37.57 11.16,38.01 11.79,38.65 11.79,40.42 11.55,40.67 R3.1 | DP.T 17.12,51.22 | 17.12,51.22 17,51.22 | 17,51.22 16.87,51.22 v16.74,51.09 | 17,51.22 17.89,51.47 | 17.12,51.22 17.7,51.6 | 17,51.22 17.63,51.09 | 17.12,51.22 17.76,50.84
  Bottom 0.152: v11.79,36.93 12.11,37.25 14.71,37.25 18.62,41.16 18.62,49.26 17.68,50.2 17,50.2 16.74,50.46 v16.74,51.09
N$7
  Top 0.152: Q1.1 11.24,40.09 11.41,39.92 11.41,38.71 10.99,38.29 R4.1 10.74,37.54 11.03,37.25 11.03,36.84 11.57,36.3 R5.1 R6.2
N$8  (via drill 0.25 pad 0.51)
  Top 0.152: R2.1 11.94,37.67 v11.79,37.82 | DM.T 17.38,49.19 | 17.12,49.19 17,49.19 | 17,49.19 16.87,49.19 v16.74,49.06 | 17.12,49.19 17.38,49.19 | 17.38,49.19 17.63,49.44 17.12,49.19 | 17.12,49.19 17.76,49.06 | 17,49.19 17.89,49.63 | 17,49.19 17.89,48.74
  Bottom 0.152: v11.79,37.82 v11.8,37.82 12.02,37.61 14.56,37.61 18.27,41.31 18.27,49.09 17.53,49.82 17,49.82 16.74,49.57 v16.74,49.06
N$9  (via drill 0.25 pad 0.51)
  Top 0.152: R7.2 12.91,41.21 v13.06,41.06 | VBUS.T 17.12,47.16 | 17.12,47.16 17,47.16 | 17,47.16 v12.93,47.16 | 17,47.16 17.82,47.6 | 17.12,47.16 17.63,47.28 | 17.12,47.16 17.63,46.9 | 17,47.16 17.82,46.71
  Bottom 0.152: v13.06,41.06 13.06,47.03 v12.93,47.16
N$10
  Top 0.152: U1.3 17.11,40.92 17.51,41.31 18.27,41.31 R8.2
N$11
  Top 0.152: 7.35,37.12 7.09,37.12
  Top 0.203: U2.5 7.06,37.79 | 7.06,37.79 7.06,37.67 | 7.06,37.67 7.35,37.38 | 7.06,37.67 7.06,37.16 7.09,37.12 | 7.06,37.79 7.35,37.5
  Top 1.016: L1.2 7.4,37.07 7.35,37.12
N$12
  Top 0.152: R13.2 2.75,42.23 3.41,41.57 4.93,41.57 5.26,41.24 U2.12
N$13
  Top 0.152: U2.10 6.16,41.23 4.96,42.43 D4.-
N$14
  Top 0.152: D4.+ 3.93,43.33 R14.2
N$15
  Top 0.152: R14.1 4.56,43.66 4.09,44.14 Q2.2
PB_5V  (via drill 0.25 pad 0.51)
  other vias: 13.7,32.23 14.33,32.36 4.68,33.31 5.31,33.31 5.95,33.31 14.08,31.79
  pour Bottom (isolate 0.254, no thermals): 14.71,31.28 9.89,31.28 8.87,32.3 4.3,32.3 4.04,32.55 4.04,33.69 4.17,33.82 9.25,33.82 10.39,32.68 14.71,32.68
  pour Top (isolate 0.254, no thermals): 4.68,32.93 6.46,32.93 6.58,33.06 6.58,34.46 6.46,34.58 4.3,34.58 4.17,34.46 4.17,33.06 4.3,32.93
  pour Top (isolate 0.254, no thermals): 12.43,28.74 14.33,28.74 14.46,28.87 14.46,30.77 14.84,31.15 14.84,33.19 14.71,33.31 14.58,33.44 14.08,33.44 13.95,33.31 13.95,32.93 13.7,32.68 12.04,31.03 11.79,30.77 11.79,28.87 11.92,28.74
PB_DATA
  Top 0.152: U4.4 9.39,34.56 R18.1 9.61,34.08 9.87,33.82 11.83,33.82 | 11.84,33.82 12.03,33.82 | D1.1 12.03,33.82 | 12.03,33.82 12.03,34.86 R19.1 | 11.83,33.82 12.02,34.02 | 11.83,33.82 11.84,33.82 | 11.84,33.82 12.02,33.64
  Top 0.305: PB_DATA.T 10.19,30.34 9.89,30.65 9.89,30.76
  Top 0.508: 10.52,29.88 10.65,29.88
  pour Top (isolate 0.254, no thermals): 9.5,29.12 10.87,29.12 11.16,29.41
  pour Top (isolate 0.254, no thermals): 10.27,28.74 9.38,28.74 9.12,28.99 9.12,30.39 9.89,31.15 11.16,32.42 11.66,32.93 11.66,33.31 11.79,33.44 12.3,33.44 12.43,33.31 12.43,32.17 11.28,31.03 11.28,28.99 11.03,28.74
PIO0_0/!RESET  (via drill 0.25 pad 0.51)
  Top 0.152: U1.2 17.61,40.79 17.76,40.93 18.39,40.93 19.09,41.63 v19.66,41.63 19.83,41.47 R11.2 20.16,42.04 C5.2 | v18.78,52.24 7.35,52.24 6.33,53.25 | SWD_!RST.T 5.82,53.25 | 5.82,53.25 5.95,53.25 | 5.95,53.25 6.08,53.25 | 6.08,53.25 6.2,53.25 | 6.2,53.25 6.33,53.25 | 6.08,53.25 5.57,53.38 | 6.08,53.25 5.31,53.51 6.2,53.25 | 6.2,53.25 5.12,53.7 6.33,53.25 | 5.82,53.25 5.44,53.12 | 6.33,53.25 5.12,52.81 | 5.95,53.25 5.57,53
  Bottom 0.152: v18.78,52.24 18.78,50.51 19.77,49.52 19.77,47.43 20.55,46.65 20.55,42.46 19.73,41.63 v19.66,41.63
PIO0_1/!ISP_EN  (via drill 0.25 pad 0.51)
  Top 0.152: R8.1 19.51,42.61 v19.54,42.58 | ISP.T 17.12,53.25 | 17.12,53.25 17,53.25 | 17.12,53.25 17.63,53.38 | 17.12,53.25 17.76,53.51 | 17.12,53.25 17.76,53.63 | 17,53.25 17.82,53.7 | 17,53.25 17.63,53.12 | 17,53.25 17.76,53 | 17,53.25 17.89,52.81 | 17,53.25 16.74,53.25 v16.68,53.19
  Bottom 0.152: v19.54,42.58 20.17,43.22 20.17,46.52 19.41,47.28 19.41,49.44 18.27,50.58 18.27,51.6 v16.68,53.19
PIO0_3/USB_VBUS
  Top 0.152: U1.9 13.72,39.63 12.7,40.65 R7.1
PIO0_4/SCL  (via drill 0.25 pad 0.51)
  Top 0.152: U1.10 13.33,39.13 v13.19,39.28 13.06,39.41 R16.2 | v10.34,71.21 10.08,70.95 arc-45 9.67,70.78 9.11,70.78 arc-45 7.62,71.4 7.14,71.87 arc-45 6.2,74.13 6.2,79.01 arc-45 8.08,83.56 8.22,83.69 arc-45 10.89,84.8 12.06,84.8 arc-45 15.41,83.41 15.68,83.15 arc-45 16.87,80.26 16.87,58.68 arc-45 16.35,57.43 16.33,57.41 arc45 15.73,55.95 15.73,55.73 arc-45 15.14,54.31 14.85,54.02 arc-45 13.6,53.51 v13.57,53.51 | v10.39,14.29 10.05,14.63 arc45 9.59,14.82 9.45,14.82 arc45 7.03,13.82 arc45 6.33,12.13 6.33,5.56 arc45 7.54,2.64 8.09,2.09 arc45 11.2,0.8 12.22,0.8 arc45 14.96,1.93 15.95,2.93 arc45 17,5.46 17,23.11 arc45 16.79,23.62 arc-45 16.49,24.34 v16.49,25.57 | v9.76,50.33 v13.57,50.33
  Bottom 0.102: J1.3 12.4,73.2 arc45 12.45,73.09 arc-45 12.51,72.93 12.51,71.92 arc-45 12.26,71.31 12.1,71.16 arc-45 11.8,71.03 10.64,71.03 arc-45 10.44,71.11 v10.34,71.21 10.27,71.29 10.27,71.93 arc-45 10.35,72.13 arc45 10.47,72.42 10.47,72.93 arc-45 10.53,73.07 10.58,73.12 arc45 10.6,73.19 J1.9 | J2.3 10.6,12.33 arc45 10.52,12.51 arc-45 10.47,12.64 10.47,12.98 arc45 10.37,13.22 arc-45 10.22,13.6 10.22,13.86 arc-45 v10.39,14.29 arc-45 10.64,14.39 11.81,14.39 arc-45 12.21,14.22 12.42,14.01 arc-45 12.53,13.76 12.53,12.69 arc-45 12.45,12.51 arc45 12.4,12.38 J2.9
  Bottom 0.152: v13.19,39.28 13.95,39.28 14.58,39.92 14.58,42.71 13.95,43.35 13.95,49.95 v13.57,50.33 v13.57,53.51 | v16.49,25.57 15.98,25.06 arc-45 14.45,24.42 12.94,24.42 arc-45 7.08,26.85 0.94,32.98 0.94,45.17 6.1,50.33 v9.76,50.33
PIO0_5/SDA  (via drill 0.25 pad 0.51)
  Top 0.152: U1.11 13.3,38.63 v13.19,38.52 13.09,38.42 R17.2 | v10.77,71.79 9.22,71.79 arc-45 8.19,72.22 7.74,72.66 arc-45 7.22,73.93 7.22,79.44 arc-45 8.46,82.43 8.81,82.78 arc-45 11.41,83.86 11.47,83.86 arc-45 14.84,82.46 arc-45 15.85,80.01 15.85,59.44 arc-45 15.25,57.98 arc45 14.71,56.68 arc-45 14.18,55.38 v13.57,54.78 | v10.72,13.63 9.21,13.63 arc45 7.76,13.03 arc45 7.35,12.02 7.35,5.73 arc45 8.32,3.38 8.79,2.92 arc45 11.44,1.82 12.03,1.82 arc45 14.44,2.82 14.82,3.19 arc45 15.98,6 15.98,21.63 arc45 15.53,22.71 15.36,22.88 arc-45 14.84,24.15 v14.84,25.57 | v9.12,49.7 12.81,49.7 12.93,49.7 14.2,49.7 v14.84,50.33
  Bottom 0.102: J1.4 12.1,73.17 arc45 12.17,73.02 arc-45 12.22,72.89 12.22,71.98 arc-45 12.01,71.47 11.94,71.4 arc-45 11.67,71.29 11.43,71.29 arc-45 11.18,71.39 v10.77,71.79 10.77,72.86 arc-45 10.83,72.99 10.87,73.03 arc45 10.9,73.12 J1.8 | J2.4 10.9,12.37 arc45 10.81,12.57 arc-45 10.72,12.79 v10.72,13.63 11.11,14.01 arc-45 11.41,14.14 11.44,14.14 arc-45 12.04,13.89 12.11,13.81 arc-45 12.3,13.36 12.3,12.72 arc-45 12.26,12.62 12.16,12.53 arc45 12.1,12.37 J2.8
  Bottom 0.152: v13.19,38.52 13.82,38.52 14.97,39.66 14.97,43.09 14.33,43.73 14.33,49.82 v14.84,50.33 14.84,53.51 v13.57,54.78 | v14.84,25.57 14.54,25.27 arc-45 13.42,24.8 13.21,24.8 arc-45 7.1,27.33 1.25,33.19 1.25,45 5.95,49.7 v9.12,49.7
PIO0_6/!USB_CONNECT
  Top 0.152: U1.15 13.17,36.63 R5.2
PIO0_10/SWCLK  (via drill 0.25 pad 0.51)
  Top 0.152: SWD_CLK.T 5.06,51.09 5.95,51.09 | v19.79,50.33 16.49,50.33 15.73,51.09 6.33,51.09 | U1.19 15.61,34.98 15.37,34.73 R9.1 15.16,34.23 v14.91,34.47 | 5.95,51.09 6.2,51.09 | 6.2,51.09 6.33,51.09 | 6.2,51.09 5.31,51.22 | 6.2,51.09 5.31,51.47 | 6.33,51.09 5.19,51.66 | 5.95,51.09 5.44,50.97 | 6.2,51.09 5.19,50.84 | 6.33,51.09 5.19,50.77
  Bottom 0.152: v14.91,34.47 18.84,38.39 19.92,38.39 20.55,39.03 20.55,41.82 20.93,42.2 20.93,46.9 20.12,47.71 20.12,50 v19.79,50.33
PIO0_15/SWDIO  (via drill 0.25 pad 0.51)
  Top 0.152: U1.25 20.03,36.13 R10.1 20.66,36 v20.68,35.98 | v21.44,48.17 15.6,48.17 14.84,48.93 6.58,48.93 | 6.58,48.93 6.46,48.93 | 6.46,48.93 6.33,48.93 | 6.33,48.93 6.08,48.93 | 6.08,48.93 5.95,48.93 | 5.95,48.93 5.31,48.93 SWD_DIO.T | 5.95,48.93 5.44,49.06 | 6.08,48.93 5.31,49.31 | 6.33,48.93 5.44,49.31 | 6.46,48.93 5.31,49.44 | 5.95,48.93 5.31,48.81 | 5.95,48.93 5.06,48.68 | 6.58,48.93 5.31,49.57
  Bottom 0.152: v20.68,35.98 20.93,35.98 21.95,37 21.95,47.41 21.44,47.92 v21.44,48.17
PIO0_18/RXD  (via drill 0.25 pad 0.51)
  Top 0.152: U1.31 19.39,39.13 v19.54,39.28 | R19.2 13.71,35.1 v13.82,35.22
  Bottom 0.152: v19.54,39.28 18.78,39.28 15.41,35.92 15.35,35.85 15.22,35.73 14.33,35.73 v13.82,35.22
PIO0_19/TXD  (via drill 0.25 pad 0.51)
  Top 0.152: U4.2 v9.89,37.69 | U1.32 19,39.63 19.28,39.92 v19.28,40.04
  Bottom 0.152: v9.89,37.69 10.2,37.69 11.54,36.36 12.55,36.36 13.06,36.87 15.85,36.87 19.03,40.04 v19.28,40.04
VBAT  (via drill 0.25 pad 0.51)
  Top 0.203: U2.2 5.71,37.51 | 5.71,37.39 5.71,36.75 5.69,36.74 5.69,36.64 5.62,36.56 | 5.71,37.51 5.71,37.39 | 5.71,37.39 5.44,37.12 | 5.71,37.51 5.31,37.12
  Top 0.305: R22.1 16.08,33.21 v16.11,33.19
  Top 0.406: U3.4 U3.3 | v9.61,71.29 9.15,71.29 arc-45 7.8,71.84 7.54,72.11 arc-45 6.71,74.1 6.71,79.1 arc-45 8.37,83.1 8.63,83.37 arc-45 11.04,84.37 11.46,84.37 arc-45 15.27,82.79 arc-45 16.36,80.16 16.36,58.94 arc-45 15.93,57.9 15.75,57.72 arc45 15.22,56.44 15.22,55.79 arc-45 14.68,54.49 arc-45 13.83,54.14 13.24,54.14 arc45 12.5,53.83 v12.17,53.51 | v9.58,14.31 9.46,14.31 arc45 7.46,13.48 arc45 6.84,11.99 6.84,5.6 arc45 7.9,3.04 8.21,2.73 arc45 11.64,1.31 12.19,1.31 arc45 14.54,2.28 15.39,3.13 arc45 16.49,5.78 16.49,22.34 arc45 16.18,23.08 15.97,23.29 arc-45 15.6,24.19 v15.6,26.2
  Top 0.508: C12.2 10.61,41.92 v10.52,42.01 10.72,42.21 U3.3
  Top 1.016: L1.1 5.62,36.56 5.44,36.74
  Bottom 0.152: J1.2 12.7,73.27 arc-45 12.81,73.02 12.81,71.8 arc-45 12.54,71.14 12.31,70.92 arc-45 11.79,70.7 10.34,70.7 arc-45 9.7,70.97 9.61,71.06 v9.61,71.29 9.61,71.59 arc-45 9.73,71.89 10.02,72.18 arc45 10.19,72.6 10.19,73.05 arc-45 10.25,73.2 10.3,73.25 J1.10 | J2.2 10.3,12.3 arc-45 10.19,12.56 10.19,12.81 arc45 10.06,13.12 9.82,13.36 arc-45 9.58,13.94 v9.58,14.31 9.88,14.61 arc-45 10.38,14.82 11.76,14.82 arc-45 12.38,14.56 12.58,14.36 arc-45 12.81,13.82 12.81,12.56 arc-45 12.7,12.3 J2.10
  Bottom 0.406: v3.79,36.93 3.85,37 4.17,37 4.36,37 v4.42,36.93 | v4.42,36.93 4.42,36.61 4.17,36.36 | v4.42,36.93 4.36,36.93 4.04,36.61 | 4.55,36.61 4.3,36.36 | 4.55,36.61 4.55,35.85 4.68,35.73 | v15.6,26.2 15.6,26.23 15.63,26.23 17.89,28.49 17.89,31.41 v16.11,33.19 | 4.55,36.61 4.55,37 4.3,37.25 | 9.5,47.41 11.31,49.22 arc45 12.17,51.29 v12.17,53.51 12.3,53.63 12.3,55.41 | 9.5,47.41 9,46.9 | 9.5,47.41 9.5,46.77 | VBAT.T 12.3,55.41 | 12.3,55.41 11.98,56.3 | 12.3,55.41 12.62,56.3
  Bottom 0.508: 3.79,36.87 3.79,36.61 4.68,35.73 6.33,34.07 14.08,34.07 14.46,33.69 15.6,33.69 v16.11,33.19 | 3.79,36.87 v3.79,36.93 | 4.17,37 4.17,37.25 | 4.17,37.25 3.79,36.87 | v10.52,42.01 10.52,42.08 10.27,42.33 10.27,46.01 9.5,46.77 9.38,46.9 9,46.9 6.08,46.9 3.66,44.49 3.66,38.65 4.17,38.14 4.17,37.25
  pour Top (isolate 0.254, no thermals): 6.08,35.34 6.08,36.74 5.57,37.25 3.33,37.25 3.15,37.07 3.15,35.34 3.28,35.22 5.95,35.22

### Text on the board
tPlace: GND | !RST | CLK | DIO | 3V3 | Seeed
bPlace: Xadow | Pebble Time Adapter | v1.0 10/06/2015
enhance: Goldfinger Area, / Torence +/-0.03mm, / Total Thickness = 0.2mm | Enhance other Area, / Torence +/-0.03mm, / Total Thickness = 0.3mm | Goldfinger Area, / Torence +/-0.03mm, / Total Thickness = 0.2mm

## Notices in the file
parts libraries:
moudle-new: This work is licensed under the Creative Commons Attribution 4.0 International License.
To view a copy of this license,visit:
http://creativecommons.org/licenses/by-sa/4.0
moudle-new: CC-BY-SA
